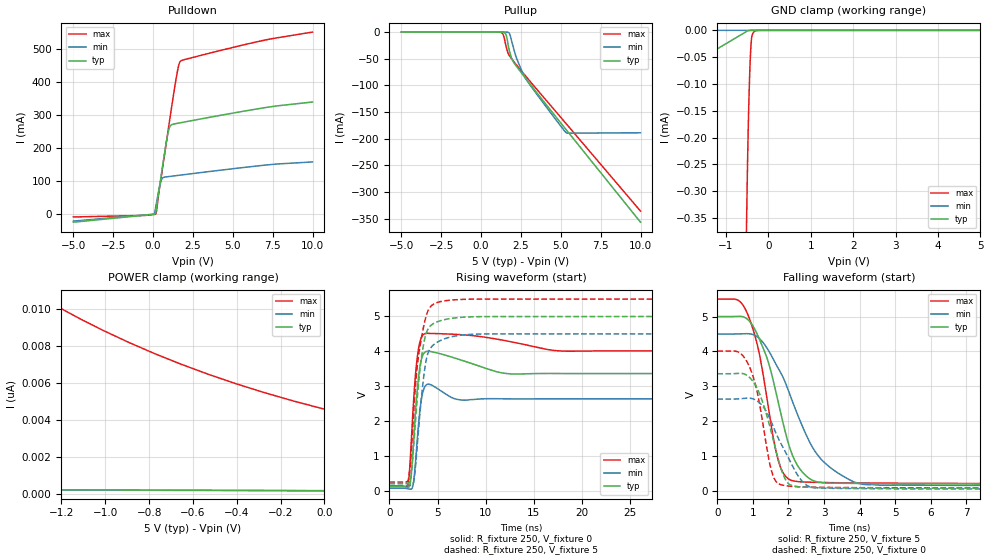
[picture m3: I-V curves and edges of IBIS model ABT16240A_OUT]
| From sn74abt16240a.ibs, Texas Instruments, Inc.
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[Model]   ABT16240A_OUT
Model_type  3-state
Enable   Active-Low
Vref =   0.0
Rref =   500
Cref =   50p
Vmeas =   1.5
| variable   typ   min   max
C_comp   5.60pF   4.59pF   8.50pF
| C_pullup   6.26pF   4.77pF   9.25pF
| C_pulldown   6.81pF   0.54pF   18.42pF
| C_tri-state   5.60pF   4.59pF   8.50pF
[Temperature Range]   40   -40   100
| Ambient temperature   25   -40   85
[Voltage range]   5   4.5   5.5
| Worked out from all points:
|   slope of the pulldown table from 0 to 0.75 V, typ, clamps not added: 3.86 ohm
|   rising waveform, R_fixture 250, V_fixture 0: 20-80 % time 480ps typ, 461ps min, 511ps max; typ from 0.122 V to 3.36 V
|   falling waveform, R_fixture 250, V_fixture 5: 20-80 % time 751ps typ, 1.18ns min, 560ps max; typ from 5 V to 0.212 V
|   rising waveform, R_fixture 250, V_fixture 5: 20-80 % time 959ps typ, 934ps min, 1.06ns max; typ from 0.212 V to 5 V
|   falling waveform, R_fixture 250, V_fixture 0: 20-80 % time 536ps typ, 728ps min, 428ps max; typ from 3.36 V to 0.122 V
[GND Clamp]
| ABT16240A_OUT
|   Voltage   I(typ)   I(min)   I(max)
-5V       -212.8uA   -82.78nA   -22.35mA
-2.49V    -95.01uA   -37.88nA   -10.05mA
-495mV    -1.366uA   -2.188nA   -277.6uA
-485mV    -997.3nA   -2.048nA   -232.9uA
-475mV    -729.8nA   -1.946nA   -193.1uA
-455mV    -392.6nA   -1.814nA   -126.7uA
-435mV    -211.1nA   -1.738nA   -75.28uA
-415mV    -112.6nA   -1.69nA    -37.78uA
-400mV    -69.93nA   -1.666nA   -19.81uA
-385mV    -43.45nA   -1.647nA   -10.18uA
-310mV    -6.516nA   -1.585nA   -1.334uA
5V        158.2pA    167.2pA    3.297nA
[POWER Clamp]
| ABT16240A_OUT
|   Voltage   I(typ)   I(min)   I(max)
-5V       371.7pA    337.6pA    120nA
-1.33V    211.7pA    196.7pA    10.89nA
-1.225V   207.4pA    192.9pA    10.17nA
-1.115V   202.9pA    189pA      9.468nA
-1.005V   198.4pA    185pA      8.812nA
-890mV    193.7pA    181pA      8.174nA
-775mV    189.1pA    176.9pA    7.583nA
-655mV    184.3pA    172.7pA    7.012nA
-530mV    179.2pA    168.2pA    6.462nA
-405mV    174.2pA    163.6pA    5.956nA
-275mV    169.1pA    158.6pA    5.471nA
-84.45fV  158.2pA    148pA      4.571nA
[Pulldown]
| ABT16240A_OUT
|   Voltage   I(typ)   I(min)   I(max)
-5V       -24.88mA   -21.51mA   -9.056mA
55mV      -942.6uA   -664.3uA   -1.465mA
165mV     3.931mA    20.39mA    402.8uA
225mV     24.2mA     37.09mA    12.07mA
530mV     123.2mA    103.7mA    118.7mA
990mV     256mA      113.4mA    268.4mA
1.135V    269.5mA    114.3mA    315.1mA
1.51V     274.4mA    116.5mA    427.6mA
1.63V     275.5mA    117.2mA    453.7mA
1.74V     276.5mA    117.9mA    463.6mA
6.645V    319.1mA    146mA      522.8mA
10V       339.1mA    157.6mA    550.8mA
[Pullup]
| ABT16240A_OUT
|   Voltage   I(typ)   I(min)   I(max)
-5V       -15pA      -12.34pA   -42.3pA
1.155V    -3.199uA   -825.2pA   -149.4uA
1.36V     -139.3uA   -109.7nA   -3.337mA
1.485V    -1.328mA   -2.379uA   -15.29mA
1.6V      -8.309mA   -40.17uA   -30.23mA
1.78V     -35.13mA   -2.674mA   -44.34mA
1.92V     -49.37mA   -17.14mA   -50.25mA
2.035V    -56.16mA   -29.87mA   -54.7mA
2.3V      -67.42mA   -54.48mA   -64.56mA
2.795V    -86.89mA   -87.03mA   -82.48mA
5.335V    -183.1mA   -188.8mA   -171.9mA
10V       -356.9mA   -189.1mA   -336.1mA
[Ramp]
| ABT16240A_OUT
| variable   typ   min   max
dV/dt_r   2.34/6.35E-10   1.81/5.86E-10   2.64/6.31E-10
dV/dt_f   2.89/7.59E-10   2.61/1.18E-09   3.17/5.67E-10
R_load = 250
[Rising Waveform]
| ABT16240A_OUT
R_fixture =   250
C_fixture =   0
L_fixture =   0
V_fixture =   0
V_fixture_min = 0
V_fixture_max = 0
|   Time   V(typ)   V(min)   V(max)
0s        122.4mV    71.78mV    139.3mV
1.93ns    99.94mV    54.18mV    170.7mV
2.255ns   416.2mV    45.85mV    1.326V
2.525ns   1.491V     291.6mV    2.627V
2.825ns   2.674V     1.223V     3.657V
3.24ns    3.665V     2.466V     4.336V
3.675ns   3.972V     2.985V     4.504V
7.215ns   3.769V     2.612V     4.481V
12.65ns   3.351V     2.635V     4.272V
50ns      3.362V     2.635V     4.01V
[Falling Waveform]
| ABT16240A_OUT
R_fixture =   250
C_fixture =   0
L_fixture =   0
V_fixture =   5
V_fixture_min = 4.5
V_fixture_max = 5.5
|   Time   V(typ)   V(min)   V(max)
0s        5V         4.5V       5.5V
645ps     5.007V     4.505V     5.419V
1.045ns   4.652V     4.466V     4.496V
1.41ns    3.77V      4.074V     2.562V
1.73ns    2.47V      3.485V     819.8mV
2.02ns    1.291V     2.822V     333.8mV
2.285ns   685.1mV    2.118V     268.4mV
2.975ns   235.2mV    851.9mV    243.7mV
4.22ns    214.7mV    180.3mV    228.8mV
50ns      211.9mV    153.7mV    249.4mV
[Rising Waveform]
| ABT16240A_OUT
R_fixture =   250
C_fixture =   0
L_fixture =   0
V_fixture =   5
V_fixture_min = 4.5
V_fixture_max = 5.5
|   Time   V(typ)   V(min)   V(max)
0s        212mV      154mV      249.6mV
1.935ns   215.8mV    150.7mV    301mV
2.215ns   356.6mV    156.2mV    903.6mV
2.49ns    1.162V     223.9mV    2.091V
2.905ns   2.703V     1.341V     3.602V
3.51ns    4.14V      3.149V     4.651V
3.975ns   4.62V      3.92V      5.142V
4.825ns   4.83V      4.237V     5.388V
9.425ns   4.995V     4.496V     5.498V
50ns      5V         4.5V       5.499V
[Falling Waveform]
| ABT16240A_OUT
R_fixture =   250
C_fixture =   0
L_fixture =   0
V_fixture =   0
V_fixture_min = 0
V_fixture_max = 0
|   Time   V(typ)   V(min)   V(max)
0s        3.362V     2.636V     4.01V
650ps     3.374V     2.646V     3.944V
1.035ns   3.094V     2.63V      3.182V
1.285ns   2.516V     2.42V      1.907V
1.565ns   1.498V     1.868V     446.5mV
1.86ns    448.7mV    1.223V     163.9mV
2.135ns   145.8mV    677.6mV    130.5mV
2.585ns   105.9mV    126.9mV    110.5mV
3.455ns   91.72mV    73.34mV    99.09mV
50ns      122.3mV    71.69mV    139.3mV
